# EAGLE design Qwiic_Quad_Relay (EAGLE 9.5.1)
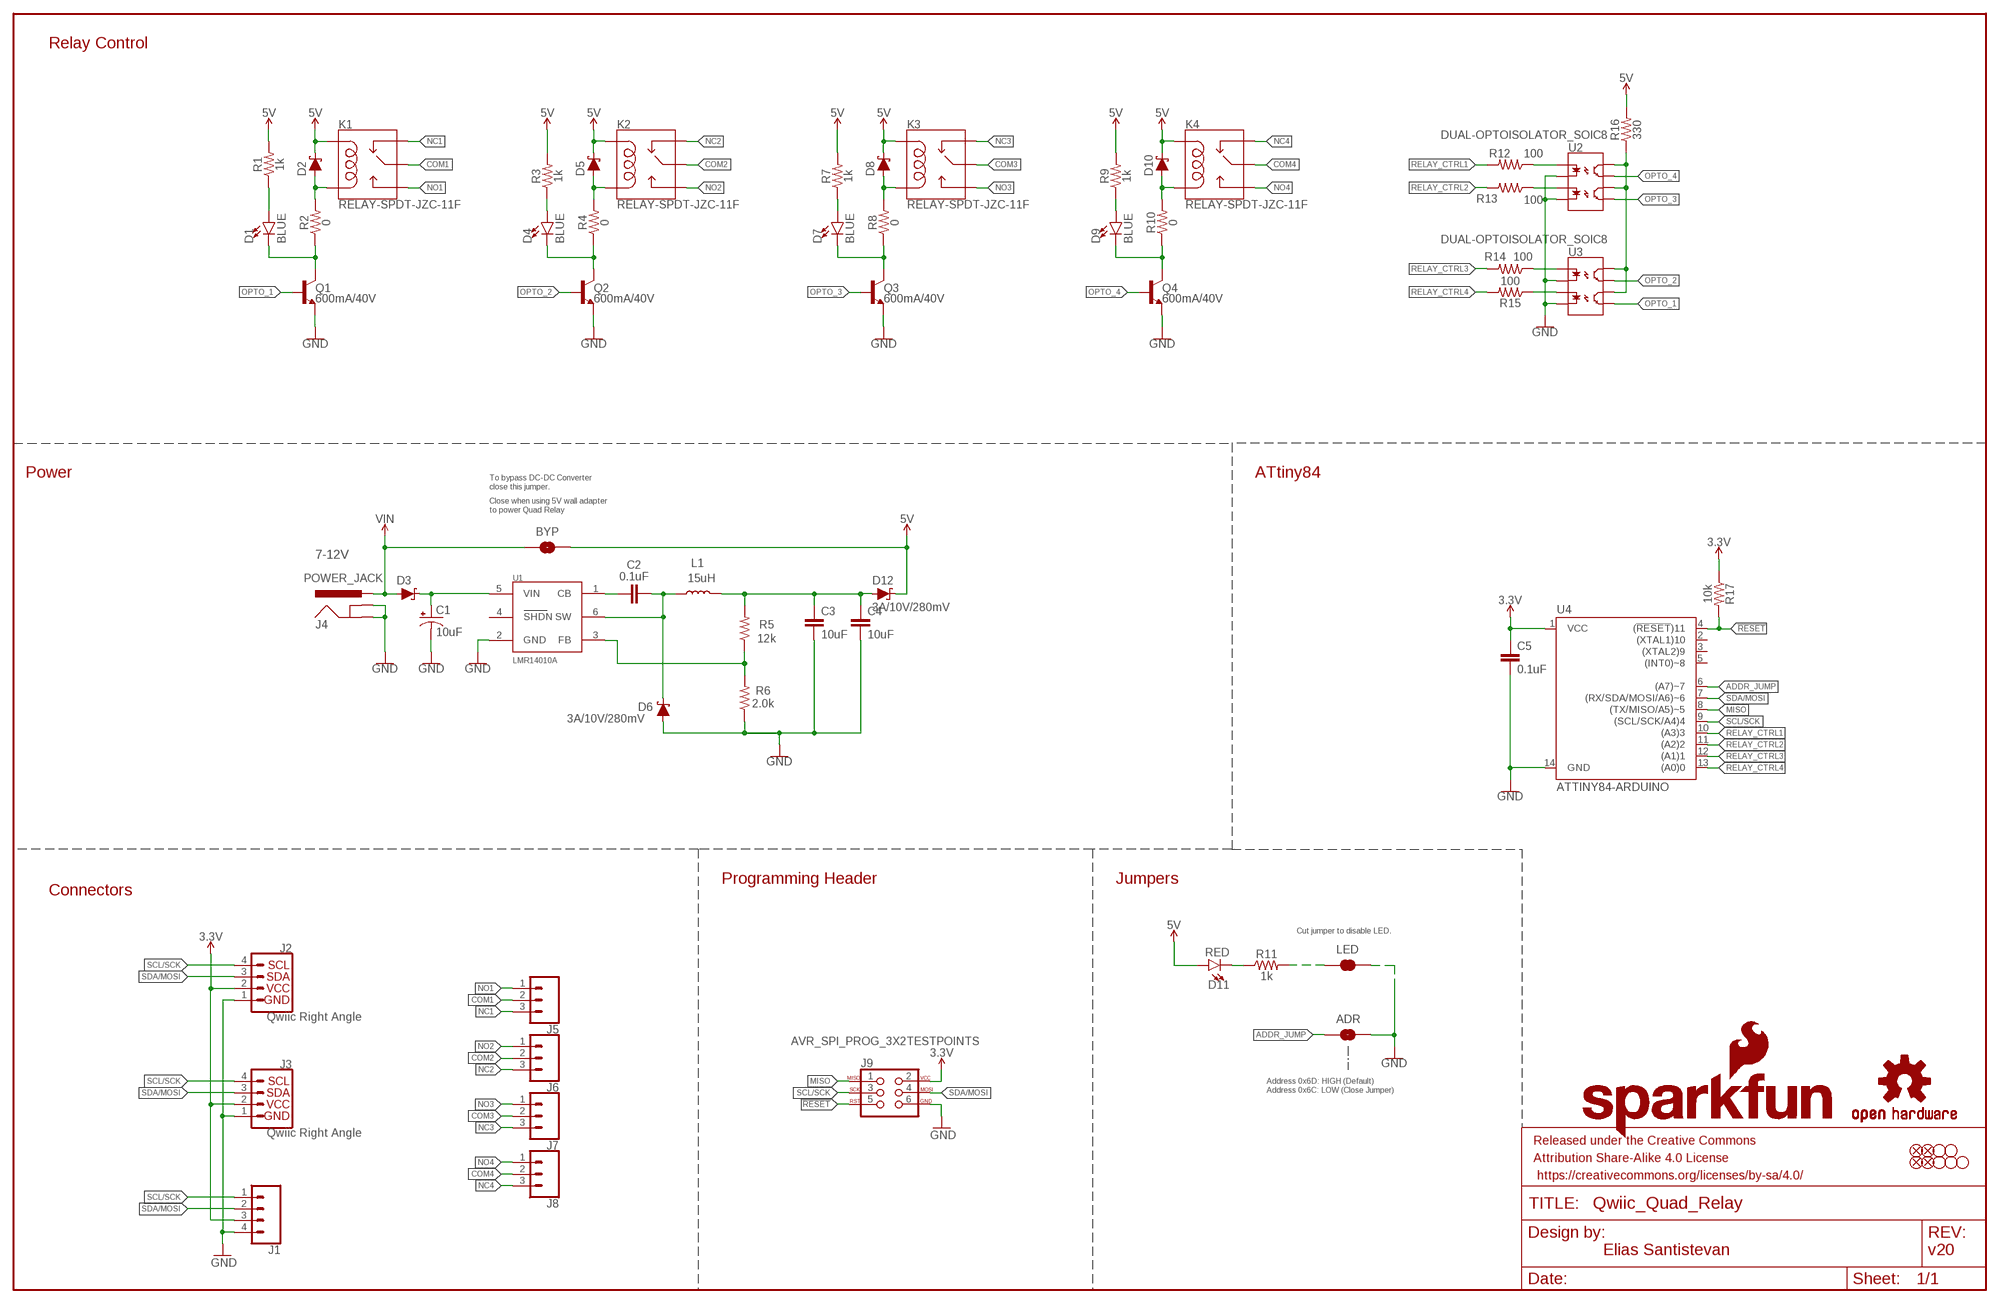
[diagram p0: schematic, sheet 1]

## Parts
ADR  JUMPER-SMT_2_NO_SILK  [SMT-JUMPER_2_NO_SILK]
BYP  JUMPER-SMT_2_NO_SILK  [SMT-JUMPER_2_NO_SILK]
C1  10uF  10UF-POLAR-EIA3528-20V-10%(TANT)  [EIA3528]
C2  0.1uF  0.1UF-0402-10V-10%-X7R  [0402]
C3  10uF  10UF-0603-6.3V-20%  [0603]
C4  10uF  10UF-0603-6.3V-20%  [0603]
C5  0.1uF  0.1UF-0603-25V-(+80/-20%)  [0603]
D1  BLUE  LED-BLUE0603  [LED-0603]
D2  1A/23V/620mV  DIODE-SCHOTTKY-BAT20J  [SOD-323]
D3  1A/40V/500mV  DIODE-SCHOTTKY-SS14  [SMA-DIODE]
D4  BLUE  LED-BLUE0603  [LED-0603]
D5  1A/23V/620mV  DIODE-SCHOTTKY-BAT20J  [SOD-323]
D6  3A/10V/280mV  DIODE-SCHOTTKY-BAT60A  [SOD-323]
D7  BLUE  LED-BLUE0603  [LED-0603]
D8  1A/23V/620mV  DIODE-SCHOTTKY-BAT20J  [SOD-323]
D9  BLUE  LED-BLUE0603  [LED-0603]
D10  1A/23V/620mV  DIODE-SCHOTTKY-BAT20J  [SOD-323]
D11  RED  LED-RED0603  [LED-0603]
D12  3A/10V/280mV  DIODE-SCHOTTKY-BAT60A  [SOD-323]
FD1  FIDUCIAL1X2  [FIDUCIAL-1X2]
FD2  FIDUCIAL1X2  [FIDUCIAL-1X2]
FD3  FIDUCIAL1X2  [FIDUCIAL-1X2]
FD4  FIDUCIAL1X2  [FIDUCIAL-1X2]
FRAME1  FRAME-LEDGER  [CREATIVE_COMMONS]
J1  CONN_041X04_NO_SILK_NO_POP  [1X04_NO_SILK]
J2  Qwiic Right Angle  I2C_STANDARDQWIIC  [JST04_1MM_RA]
J3  Qwiic Right Angle  I2C_STANDARDQWIIC  [JST04_1MM_RA]
J4  POWER_JACK  [POWER_JACK_PTH]
J5  CONN_03-SCREW-5MM  [SCREWTERMINAL-5MM-3]
J6  CONN_03-SCREW-5MM  [SCREWTERMINAL-5MM-3]
J7  CONN_03-SCREW-5MM  [SCREWTERMINAL-5MM-3]
J8  CONN_03-SCREW-5MM  [SCREWTERMINAL-5MM-3]
J9  AVR_SPI_PROG_3X2TESTPOINTS  [2X3_TEST_POINTS]
JP1  STAND-OFF  [STAND-OFF]
JP4  STAND-OFF  [STAND-OFF]
JP5  STAND-OFF  [STAND-OFF]
JP6  STAND-OFF  [STAND-OFF]
JP7  STAND-OFF  [STAND-OFF]
K1  RELAY-SPDT-JZC-11F  [RELAY-JZC]
K2  RELAY-SPDT-JZC-11F  [RELAY-JZC]
K3  RELAY-SPDT-JZC-11F  [RELAY-JZC]
K4  RELAY-SPDT-JZC-11F  [RELAY-JZC]
L1  15uH  INDUCTOR-LQH5B-15UH  [INDUCTOR_15UH]
LED  JUMPER-SMT_2_NC_TRACE_SILK  [SMT-JUMPER_2_NC_TRACE_SILK]
LOGO1  SFE_LOGO_NAME_FLAME.1_INCH  [SFE_LOGO_NAME_FLAME_.1]
LOGO2  OSHW-LOGOS  [OSHW-LOGO-S]
Q1  600mA/40V  TRANS_NPN-MMBT2222AL  [SOT23-3]
Q2  600mA/40V  TRANS_NPN-MMBT2222AL  [SOT23-3]
Q3  600mA/40V  TRANS_NPN-MMBT2222AL  [SOT23-3]
Q4  600mA/40V  TRANS_NPN-MMBT2222AL  [SOT23-3]
R1  1k  1KOHM-0603-1/10W-1%  [0603]
R2  0  0OHM-0603-1/10W  [0603]
R3  1k  1KOHM-0603-1/10W-1%  [0603]
R4  0  0OHM-0603-1/10W  [0603]
R5  12k  12KOHM-0603-1/10W-1%  [0603]
R6  2.0k  2.0KOHM-0603-1/10W-5%  [0603]
R7  1k  1KOHM-0603-1/10W-1%  [0603]
R8  0  0OHM-0603-1/10W  [0603]
R9  1k  1KOHM-0603-1/10W-1%  [0603]
R10  0  0OHM-0603-1/10W  [0603]
R11  1k  1KOHM-0603-1/10W-1%  [0603]
R12  100  100OHM-0603-1/10W-1%  [0603]
R13  100  100OHM-0603-1/10W-1%  [0603]
R14  100  100OHM-0603-1/10W-1%  [0603]
R15  100  100OHM-0603-1/10W-1%  [0603]
R16  330  330OHM-0603-1/10W-1%  [0603]
R17  10k  10KOHM-0603-1/10W-1%  [0603]
U1  LMR14010A  [SOT23-6]
U2  DUAL-OPTOISOLATOR_SOIC8  [SO08]
U3  DUAL-OPTOISOLATOR_SOIC8  [SO08]
U4  ATTINY84-ARDUINO  [SO14]

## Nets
3.3V: C5.1 J1.3 J2.2 J3.2 J9.2 R17.1 U4.1(VCC)
5V: BYP.2 D2.C D5.C D8.C D10.C D11.A D12.C K1.5(COIL1) K2.5(COIL1) K3.5(COIL1) K4.5(COIL1) R1.2 R3.2 R7.2 R9.2 R16.2
5V_OUT: C3.1 C4.1 D12.A L1.P2 R5.2
!RESET: J9.5 R17.2 U4.4((!RESET!)11)
ADDR_JUMP: ADR.1 U4.6((A7)~7)
CB: C2.1 U1.1(CB)
COM1: J5.2 K1.4(MAIN)
COM2: J6.2 K2.4(MAIN)
COM3: J7.2 K3.4(MAIN)
COM4: J8.2 K4.4(MAIN)
FB: R5.1 R6.2 U1.3(FB)
GND: ADR.2 C1.C(-) C3.2 C4.2 C5.2 D6.A J1.4 J2.1 J3.1 J4.GND J4.GNDBREAK J9.6 LED.1 Q1.2(E) Q2.2(E) Q3.2(E) Q4.2(E) R6.1 U1.2(GND) U2.2(C1) U2.4(C2) U3.2(C1) U3.4(C2) U4.14(GND)
MISO: J9.1 U4.8((TX/MISO/A5)~5)
N$1: D1.A R1.1
N$2: D1.C Q1.3(C) R2.1
N$3: R15.1 U3.3(A2)
N$4: D4.A R3.1
N$5: R14.1 U3.1(A1)
N$6: R16.1 U2.6(CL2) U2.8(CL1) U3.6(CL2) U3.8(CL1)
N$7: D7.A R7.1
N$8: D9.A R9.1
N$9: R12.1 U2.1(A1)
N$10: D2.A K1.1(COIL2) R2.2
N$11: R13.1 U2.3(A2)
N$12: D4.C Q2.3(C) R4.1
N$13: D11.C R11.1
N$14: LED.2 R11.2
N$15: D7.C Q3.3(C) R8.1
N$17: D9.C Q4.3(C) R10.1
N$18: D5.A K2.1(COIL2) R4.2
N$23: D8.A K3.1(COIL2) R8.2
N$24: D10.A K4.1(COIL2) R10.2
NC1: J5.3 K1.2(NC)
NC2: J6.3 K2.2(NC)
NC3: J7.3 K3.2(NC)
NC4: J8.3 K4.2(NC)
NO1: J5.1 K1.3(NO)
NO2: J6.1 K2.3(NO)
NO3: J7.1 K3.3(NO)
NO4: J8.1 K4.3(NO)
OPTO_1: Q1.1(B) U3.5(EM2)
OPTO_2: Q2.1(B) U3.7(EM1)
OPTO_3: Q3.1(B) U2.5(EM2)
OPTO_4: Q4.1(B) U2.7(EM1)
RELAY_CTRL1: R12.2 U4.10((A3)3)
RELAY_CTRL2: R13.2 U4.11((A2)2)
RELAY_CTRL3: R14.2 U4.12((A1)1)
RELAY_CTRL4: R15.2 U4.13((A0)0)
SCL/SCK: J1.1 J2.4 J3.4 J9.3 U4.9((SCL/SCK/A4)4)
SDA/MOSI: J1.2 J2.3 J3.3 J9.4 U4.7((RX/SDA/MOSI/A6)~6)
SW: C2.2 D6.C L1.P1 U1.6(SW)
VIN: BYP.1 D3.A J4.PWR
VIN_DC_DC: C1.A(+) D3.C U1.5(VIN)
Unconnected: U1.4(SHDN) U4.2((XTAL1)10) U4.3((XTAL2)9) U4.5((INT0)~8)

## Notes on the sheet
- Relay Control
- Power | ATtiny84
- To bypass DC-DC Converter
  close this jumper.
- Close when using 5V wall adapter
  to power Quad Relay
- 7-12V
- Programming Header | Jumpers
- Connectors
- Cut jumper to disable LED.
- Address 0x6D: HIGH (Default)
  Address 0x6C: LOW (Close Jumper)
- Elias Santistevan | v20

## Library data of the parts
ADR BYP = SparkFun-Jumpers:JUMPER-SMT_2_NO: Normally open jumper
C1 = SparkFun-Capacitors:10UF-POLAR: 10.0µF polarized capacitors; PROD_ID: CAP-08063
C2 = SparkFun-Capacitors:0.1UF: 0.1µF ceramic capacitors; PROD_ID: CAP-15083
C3 C4 = SparkFun-Capacitors:10UF: 10.0µF ceramic capacitors; PROD_ID: CAP-11015
C5 = SparkFun-Capacitors:0.1UF: 0.1µF ceramic capacitors; PROD_ID: CAP-00810
D1 D4 D7 D9 = SparkFun-LED:LED-BLUE: Blue SMD LED; PROD_ID: DIO-08575
D2 D5 D8 D10 = SparkFun-DiscreteSemi:DIODE-SCHOTTKY: Schottky diode; PROD_ID: DIO-11623
D3 = SparkFun-DiscreteSemi:DIODE-SCHOTTKY: Schottky diode; PROD_ID: DIO-08053
D6 D12 = SparkFun-DiscreteSemi:DIODE-SCHOTTKY: Schottky diode; PROD_ID: DIO-14072
D11 = SparkFun-LED:LED-RED: Red SMD LED; PROD_ID: DIO-00819
FD1-FD4 = SparkFun-Aesthetics:FIDUCIAL: Fiducial Alignment Points
FRAME1 = SparkFun-Aesthetics:FRAME-LEDGER: Schematic Frame - Ledger
J1 = SparkFun-Connectors:CONN_04: Multi connection point. Often used as Generic Header-pin footprint for 0.1 inch spaced/style header connections On any of the 0.1 inch spaced packages, you can populate with these: Break Away Headers - Straight (PRT-00116) Break Away Male Headers - Right Angle (PRT-00553) Female Headers (PRT-00115)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
J2 J3 = SparkFun-Connectors:I2C_STANDARD: SparkFun I2C Standard Pinout Header SparkFun has standardized on a pinout for all I2C based sensor breakouts. This pinout allows I2C boards to be plugged directly into the headers on Arduino Uno compatible boards, and to be daisy chained easily. Example SparkFun Products: SparkFun Atmospheric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; PROD_ID: CONN-13694
J4 = SparkFun-Connectors:POWER_JACK: Power Jack Connector This is the standard 5.5mm barrel jack for power. The PTH is the most common, proven, reliable, footprint. The Slot footprint only works if the mill layer is transmitted to the PCB fab house so be warned. Here are the connectors we sell at SparkFun: DC Barrel Power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; PROD_ID: CONN-08197
J5-J8 = SparkFun-Connectors:CONN_03: Multi connection point. Often used as Generic Header-pin footprint for 0.1 inch spaced/style header connections On any of the 0.1 inch spaced packages, you can populate with these: Break Away Headers - Straight (PRT-00116) Break Away Male Headers - Right Angle (PRT-00553) Female Headers (PRT-00115)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; PROD_ID: CONN-10134; SF_SKU: PRT-08433
J9 = SparkFun-Connectors:AVR_SPI_PROG_3X2: AVR ISP 6 Pin This is the reduced ISP connector for AVR programming. Common on Arduino. This footprint will take up less PCB space and can be used with a 10-pin to 6-pin adapter such as SKU: BOB-08508 **Special note about "TEST_POINT" package. The stop mask is on the top side, so if you want your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
JP1 JP4-JP7 = SparkFun-Hardware:STAND-OFF: Stand Off
K1-K4 = SparkFun-Electromechanical:RELAY-SPDT: SPDT Electromechanical Relay Single-pole, double-throw sealed relays. When current is applied to the coil, it throws a simple changeover switch, terminating the connection from the NC contact to ground and closing the NO contact. Use them to switch high voltage/high current devices. SparkFun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; PROD_ID: COMP-09533; SF_SKU: COM-00100
L1 = SparkFun-Coils:INDUCTOR: Inductors; PROD_ID: NDUC-15090
LED = SparkFun-Jumpers:JUMPER-SMT_2_NC_TRACE: Normally closed trace jumper
LOGO1 = SparkFun-Aesthetics:SFE_LOGO_NAME_FLAME: SparkFun Font Logo w/ Flame
LOGO2 = SparkFun-Aesthetics:OSHW-LOGO: Open-Source Hardware (OSHW) Logo
Q1-Q4 = SparkFun-DiscreteSemi:TRANS_NPN: NPN transistor Current controlled devices typically used to amplify current or used as a switch. BC547 - COM-08928 (TO-92 45V 100mA) (1.Collector 2.Base 3.Emitter) 2N3904 - COM-00521 (TO-92 40V 200mA) (1.Emitter 2.Base 3.Collector) P2N2222A - COM-12852 (TO-92 40V 600mA) (1.Collector 2.Base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; PROD_ID: TRANS-08049
R1 R3 R7 R9 R11 = SparkFun-Resistors:1KOHM: 1kΩ resistor; PROD_ID: RES-07856
R2 R4 R8 R10 = SparkFun-Resistors:0OHM: 0Ω resistor; PROD_ID: RES-08609
R5 = SparkFun-Resistors:12KOHM: 12kΩ resistor; PROD_ID: RES-10327
R6 = SparkFun-Resistors:2.0KOHM: 2kΩ resistor; PROD_ID: RES-08296
R12-R15 = SparkFun-Resistors:100OHM: 100Ω resistor; PROD_ID: RES-07863
R16 = SparkFun-Resistors:330OHM: 330Ω resistor; PROD_ID: RES-00818
R17 = SparkFun-Resistors:10KOHM: 10kΩ resistor; PROD_ID: RES-00824
U1 = SparkFun-IC-Power:LMR14010A: LMR14010A Buck Regulator 1A Output The LMR14010A is a PWM DC-to-DC buck (stepdown) regulator. With a wide input range from 4 V to 40 V, it is suitable for a wide range of applications from industrial to automotive. An ultra-low 1-µA shutdown current prolongs battery life. Operating frequency is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; PROD_ID: IC-15089
U2 U3 = SparkFun-DiscreteSemi:DUAL-OPTOISOLATOR: Optocoupler, Phototransistor Output, Dual Channel Optically coupled pairs with a gallium arsenide infrared LED and a silicon NPN phototransistor. Signal information, including a DC level, can be transmitted by the device while maintaining a high degree of electrical isolation between input and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; PROD_ID: IC-09076
U4 = SparkFun-IC-Microcontroller:ATTINY84-ARDUINO; PROD_ID: IC-14155

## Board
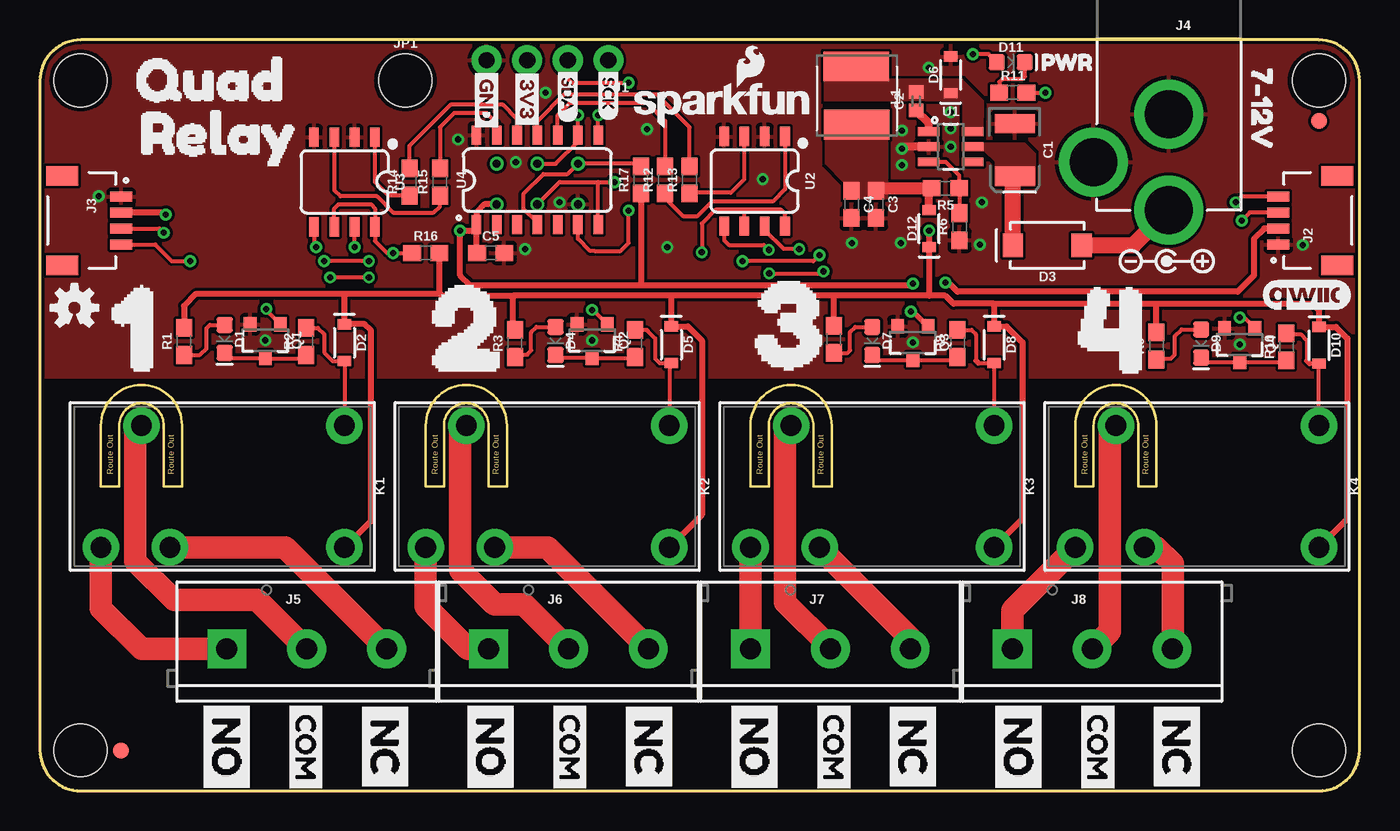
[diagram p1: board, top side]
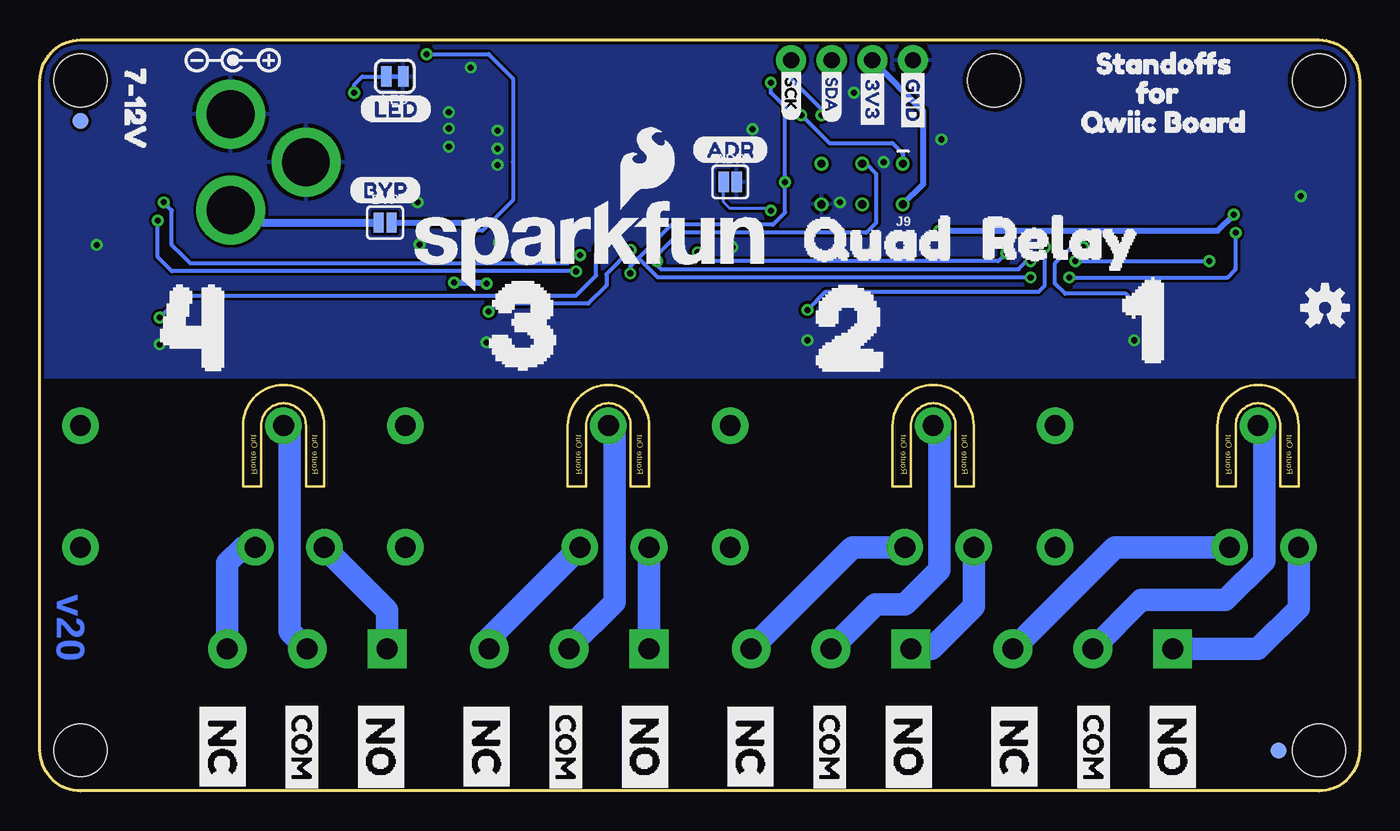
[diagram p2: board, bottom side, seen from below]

Size 82.55 x 46.99 mm. Coordinates in mm from the lower left corner, seen from the top.
Outline: 80.01,46.99 2.54,46.99 arc90 0,44.45 0,2.54 arc90 2.54,0 80.01,0 arc90 82.55,2.54 82.55,44.45 arc90 80.01,46.99
Outline: 28.07,19.05 28.07,22.86 arc90 26.67,24.26 arc90 25.27,22.86 25.27,19.05 24.13,19.05 24.13,22.86 arc-90 26.67,25.4 arc-90 29.21,22.86 29.21,19.05 28.07,19.05
Outline: 7.75,19.05 7.75,22.86 arc90 6.35,24.26 arc90 4.95,22.86 4.95,19.05 3.81,19.05 3.81,22.86 arc-90 6.35,25.4 arc-90 8.89,22.86 8.89,19.05 7.75,19.05
Outline: 48.39,19.05 48.39,22.86 arc90 46.99,24.26 arc90 45.59,22.86 45.59,19.05 44.45,19.05 44.45,22.86 arc-90 46.99,25.4 arc-90 49.53,22.86 49.53,19.05 48.39,19.05
Outline: 68.71,19.05 68.71,22.86 arc90 67.31,24.26 arc90 65.91,22.86 65.91,19.05 64.77,19.05 64.77,22.86 arc-90 67.31,25.4 arc-90 69.85,22.86 69.85,19.05 68.71,19.05
Copper layers (1*16): Top 0.035mm / dielectric 1.5mm / Bottom 0.035mm
Design rules "SparkFun-2-layer-TIGHT": minimum track width 7mil, minimum drill 15mil, track to track 7mil, track to pad 7mil, pad to pad 7mil, via to via 7mil, smd to smd 7mil, copper to edge 7mil, drill to drill 7mil, minimum pad ring 7mil, minimum via ring 7mil, stop-mask expansion 4mil, vias tented up to drill 25mil, thermal gap 10mil

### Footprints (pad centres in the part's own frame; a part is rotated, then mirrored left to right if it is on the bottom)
SMT-JUMPER_2_NO_SILK = smd 0.635 x 1.27: 1 -0.406,0; 2 0.406,0
EIA3528 = smd 1.2 x 2.5: A 1.65,0; C -1.65,0
0402 = smd 0.85 x 0.9: 1 -0.58,0; 2 0.58,0
0603 = smd 1.1 x 1: 1 -0.85,0; 2 0.85,0
LED-0603 = smd 1 x 1: A -0.877,0; C 0.877,0
SOD-323 = smd 0.63 x 0.83: A 1.15,0; C -1.15,0
SMA-DIODE = smd 1.27 x 1.47: A -2.15,0; C 2.15,0
FIDUCIAL-1X2 = smd 1 x 1: 1 0,0
1X04_NO_SILK = drill 1.016 pad 1.88: 1 0,0; 2 2.54,0; 3 5.08,0; 4 7.62,0
JST04_1MM_RA = smd 0.6 x 1.35: 1 -1.5,0; 2 -0.5,0; 3 0.5,0; 4 1.5,0 | smd 1.2 x 2: NC1 2.8,-3.675; NC2 -2.8,-3.675
POWER_JACK_PTH = drill 2.997 pad 4.318: GND 0,7.7; GNDBREAK 4.7,10.7; PWR 0,13.7
SCREWTERMINAL-5MM-3 = drill 1.3 pad 2.413 square: 1 0,0 | drill 1.3 pad 2.413: 2 5,0; 3 10,0
2X3_TEST_POINTS = drill 0.508: 1 -2.54,-1.27; 2 -2.54,1.27; 3 0,-1.27; 4 0,1.27; 5 2.54,-1.27; 6 2.54,1.27
STAND-OFF = hole 3.302: 0,0
RELAY-JZC = drill 1.3 pad 2.286: 1 3.81,-8.89; 2 -3.81,2.032; 3 -3.81,6.35; 4 3.81,3.81; 5 -3.81,-8.89
INDUCTOR_15UH = smd 1.85 x 4.1: P1 -1.905,0; P2 1.745,0.05
SMT-JUMPER_2_NC_TRACE_SILK = smd 0.66 x 1.27: 1 -0.521,0; 2 0.521,0
SOT23-3 = smd 0.8 x 0.9: 1 -0.95,-1; 2 0.95,-1; 3 0,1.1
SOT23-6 = smd 0.55 x 1.35: 1 -0.95,-1.375; 2 0,-1.375; 3 0.95,-1.375; 4 0.95,1.375; 5 0,1.375; 6 -0.95,1.375
SO08 = smd 0.6 x 1.2: 1 -1.905,-2.8; 2 -0.635,-2.8; 3 0.635,-2.8; 4 1.905,-2.8; 5 1.905,2.8; 6 0.635,2.8; 7 -0.635,2.8; 8 -1.905,2.8
SO14 = smd 0.6 x 1.2: 1 -3.81,-2.8; 2 -2.54,-2.8; 3 -1.27,-2.8; 4 0,-2.8; 5 1.27,-2.8; 6 2.54,-2.8; 7 3.81,-2.8; 8 3.81,2.8; 9 2.54,2.8; 10 1.27,2.8; 11 0,2.8; 12 -1.27,2.8; 13 -2.54,2.8; 14 -3.81,2.8

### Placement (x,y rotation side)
ADR  39.37,38.1 0 bottom
BYP  60.96,35.56 0 bottom
C1  60.99,40.11 270 top
C2  54.81,43.15 90 top
C3  52.3,36.7 270 top
C4  50.77,36.7 270 top
C5  28.19,33.66 0 top
D1  11.56,28.28 270 top
D2  19.05,28.05 270 top
D3  63.02,34.14 180 top
D4  32.26,28.16 270 top
D5  39.5,27.92 270 top
D6  56.97,44.81 90 top
D7  52.07,28.16 270 top
D8  59.69,27.92 270 top
D9  72.64,28 270 top
D10  80.01,27.89 270 top
D11  60.73,45.59 0 top
D12  55.63,35.18 90 top
FD1  80.01,41.91 0 bottom
FD2  5.08,2.54 0 top
FD3  5.08,2.54 0 bottom
FD4  80.01,41.91 0 top
FRAME1  not placed on the board
J1  35.56,45.72 180 top
J2  77.47,35.69 90 top
J3  5.08,35.69 270 top
J4  70.61,50.04 180 top
J5  11.68,8.89 0 top
J6  28.07,8.89 0 top
J7  44.45,8.89 0 top
J8  60.83,8.89 0 top
J9  31.11,37.97 180 bottom
JP1  22.86,44.45 0 top
JP4  2.54,44.45 0 top
JP5  80.01,44.45 0 top
JP6  2.54,2.54 0 top
JP7  80.01,2.54 0 top
K1  10.16,19.05 90 top
K2  30.48,19.05 90 top
K3  50.8,19.05 90 top
K4  71.12,19.05 90 top
L1  51.05,43.43 270 top
LED  60.35,44.7 180 bottom
LOGO1  42.72,42.93 0 top
LOGO2  2.16,30.23 0 top
Q1  14.1,28.19 180 top
Q2  34.54,28.19 180 top
Q3  54.61,28.07 180 top
Q4  75.06,27.94 180 top
R1  9.02,28.13 90 top
R2  16.64,28.13 90 top
R3  29.72,28 90 top
R4  37.21,28 90 top
R5  56.64,37.72 180 top
R6  57.53,35.31 90 top
R7  49.66,28.25 90 top
R8  57.4,28 90 top
R9  69.85,27.84 90 top
R10  77.98,27.78 90 top
R11  60.86,43.69 0 top
R12  39.12,38.23 90 top
R13  40.64,38.23 90 top
R14  23.11,38.1 90 top
R15  25.02,38.1 90 top
R16  24.13,33.66 0 top
R17  37.59,38.23 90 top
U1  56.97,40.31 270 top
U2  44.7,38.15 180 top
U3  19.05,38.1 180 top
U4  31.11,38.23 0 top
U$1  [7#12V0]  76.45,46.35 270 top
U$2  [20]  19.94,28.96 0 top
U$3  [10]  -0.13,28.96 0 top
U$4  [30]  40.13,29.21 0 top
U$5  [40]  60.33,28.83 0 top
U$6  [QUAD0]  3.66,44.5 0 top
U$7  [RELAY0]  4.04,41.15 0 top
U$8  [SCK-[)-03]  35.56,45.34 270 top
U$9  [GND-03]  27.94,45.34 270 top
U$10  [3V3-03]  30.48,45.34 270 top
U$11  [SDA0]  33.02,45.34 270 top
U$12  [3V3-03]  30.48,45.34 270 bottom
U$13  [OSHW-LOGO-S]  2.16,30.23 0 bottom
U$14  [BYP]  63.25,37.59 0 bottom
U$15  [NO0]  11.68,6.22 270 top
U$16  [COM0]  16.64,5.97 270 top
U$17  [NC0]  21.59,6.1 270 top
U$18  [NO0]  28.19,6.22 270 top
U$19  [COM0]  33.15,5.97 270 top
U$20  [NC0]  38.1,6.1 270 top
U$21  [NO0]  44.7,6.22 270 top
U$22  [COM0]  49.66,5.97 270 top
U$23  [NC0]  54.61,6.1 270 top
U$24  [NO0]  61.21,6.22 270 top
U$25  [COM0]  66.17,5.97 270 top
U$26  [NC0]  71.12,6.1 270 top
U$27  [NO0]  44.7,6.22 270 bottom
U$28  [COM0]  66.17,5.97 270 bottom
U$29  [NC0]  71.12,6.1 270 bottom
U$30  [NO0]  61.21,6.22 270 bottom
U$31  [COM0]  49.66,5.97 270 bottom
U$32  [NC0]  54.61,6.1 270 bottom
U$33  [NO0]  28.19,6.22 270 bottom
U$34  [COM0]  33.15,5.97 270 bottom
U$35  [NC0]  38.1,6.1 270 bottom
U$36  [NO0]  11.68,6.22 270 bottom
U$37  [COM0]  16.64,5.97 270 bottom
U$38  [NC0]  21.59,6.1 270 bottom
U$39  [10]  19.43,29.46 0 bottom
U$40  [20]  38.61,28.96 0 bottom
U$41  [30]  59.05,29.21 0 bottom
U$42  [40]  79.63,28.99 0 bottom
U$43  [QUAD0]  37.13,34.54 0 bottom
U$44  [RELAY0]  25.86,34.59 0 bottom
U$45  [GND-03]  27.94,45.34 270 bottom
U$46  [PWR_TO]  61.72,45.59 0 top
U$47  [SDA0]  33.02,45.34 270 bottom
U$48  [SCK-[)-03]  35.56,45.34 270 bottom
U$49  [7#12V0]  76.58,46.35 270 bottom
U$50  [STANDOFFS0]  17.63,45.52 0 bottom
U$51  [POLARITY_MARKING_CENTER_POSITIVE#JPG]  70.48,33.15 0 top
U$52  [FOR1]  15.14,43.69 0 bottom
U$53  [LED]  62.59,42.67 0 bottom
U$54  [POLARITY_MARKING_CENTER_POSITIVE#JPG]  70.48,45.72 0 bottom
U$55  [QWIIC_5.5MM]  79.25,31.04 0 top
U$56  [ADR-()-04]  41.78,40.13 0 bottom
U$57  [SFE_LOGO_NAME_FLAME_.2]  48.11,34.14 0 bottom
U$58  [QWIIC_BOARD2]  18.54,41.86 0 bottom

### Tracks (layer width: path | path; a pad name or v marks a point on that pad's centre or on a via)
3.3V  (via drill 0.38)
  Top 0.381: J2.2 76.59,35.19 75.95,34.54 75.95,32.26 74.93,31.24 57.4,31.24 56.84,31.8 v56.64,31.8 | v54.61,31.75 54.48,31.62 37.59,31.62 | R17.1 37.59,31.62 | 37.59,31.62 26.92,31.62 26.29,32.26 v26.29,35.05 27.3,35.05 | J9.2 27.81,36.7 27.3,36.2 U4.1 27.3,35.05 | C5.1 27.3,33.69 27.3,35.05 | v7.87,36.07 7.75,36.19 J3.2
  Bottom 0.381: v7.87,36.07 8.89,35.05 v26.29,35.05 | J9.2 28.55,36.7 27.3,37.95 27.3,42.55 J1.3 | v56.64,31.8 54.66,31.8 v54.61,31.75
5V  (via drill 0.38)
  Top 0.254: v58.37,46.1 59.35,46.1 D11.A
  Top 0.381: 49.66,30.99 39.5,30.99 | 39.5,30.99 29.59,30.99 | 59.69,30.48 57.15,30.48 56.64,30.99 55.63,30.99 | 19.05,31.11 9.78,31.11 9.02,30.35 R1.2 | 19.05,31.11 25.02,31.11 | 29.59,30.99 25.15,30.99 25.02,31.11 | D2.C | D2.C 19.05,31.11 | K1.5 20.7,16.89 20.7,28.83 20.32,29.21 D2.C | 59.69,30.48 D8.C 60.46,29.07 61.47,28.07 61.47,17.02 K3.5 | 39.5,30.99 D5.C 40.52,29.07 41.4,28.19 41.4,17.27 K2.5 | R7.2 49.66,30.99 | 59.69,30.48 69.85,30.48 | 69.85,30.48 79.63,30.48 80.01,30.1 D10.C 81.07,29.04 81.79,28.32 81.79,17.02 K4.5 | R9.2 69.85,30.48 | R16.2 24.98,31.15 25.02,31.11 | R3.2 29.59,28.98 29.59,30.99 | 55.63,30.99 49.66,30.99 | 55.63,30.99 D12.C v55.63,35.05
  Bottom 0.254: v58.37,46.1 54.48,46.1 52.96,44.58 52.96,39.37 52.96,36.96 54.86,35.05 v55.63,35.05
  Bottom 0.381: BYP.2 56.13,35.56 v55.63,35.05
5V_OUT
  Top 0.508: D12.A 55.63,37.55 R5.2
  Top 0.762: R5.2 55.75,37.68 52.43,37.68 C3.1
  pour Top (isolate 0.305, no thermals): 49.12,42.55 49.12,39.27 50.29,38.1 50.29,37.08 53.01,37.08 53.01,42.55
!RESET
  Top 0.254: R17.2 37.43,39.24 J9.5 33.02,38.61 31.5,38.61 30.23,37.34 30.23,36.44 31.11,35.55 U4.4
ADDR_JUMP  (via drill 0.38)
  Top 0.254: U4.6 33.66,34.54 34.42,33.78 34.69,33.78 36.32,33.78 36.83,34.29 v36.83,36.32
  Bottom 0.203: v36.83,36.32 36.96,36.45 39.37,36.45 39.78,36.85 ADR.1
CB
  Top 0.508: U1.1 55.6,41.79 C2.1
COM1
  Top 1.397: J5.2 16.64,8.89 13.59,11.94 8.89,11.94 8.38,11.94 5.97,14.35 5.97,22.48 K1.4
  Bottom 1.397: J5.2 13.64,11.94 8.38,11.94 5.97,14.35 5.97,22.48 K1.4
COM2
  Top 1.397: J6.2 30.27,11.68 28.45,11.68 26.29,13.84 26.29,22.48 K2.4
  Bottom 1.397: J6.2 30.27,11.68 28.45,11.68 26.29,13.84 26.29,22.48 K2.4 | J6.2
COM3
  Top 1.397: J7.2 49.45,8.97 46.61,11.81 46.61,22.48 K3.4
  Bottom 1.397: J7.2 49.45,8.97 46.61,11.81 46.61,22.48 K3.4
COM4
  Top 1.397: K4.4 66.93,22.48 66.93,9.99 J8.2
  Bottom 1.397: K4.4 66.93,22.48 66.93,9.99 J8.2
FB
  Top 0.254: U1.3 56.65,39.36 57.49,38.52 R5.1 57.53,37.68 R6.2
GND  (via drill 0.38)
  Top 0.508: U1.2 54.05,40.31 v53.92,40.18
  other vias: 30.35,33.91 39.24,34.04 37.97,41.4 50.8,34.29 45.21,38.28 31.62,43.69 29.77,39.34 26.16,40.77 32.51,36.83 34.54,28.19 14.1,28.19 54.61,28.07 75.06,27.94 53.92,39.17 58.8,34.19 55.6,45.26 78.99,34.16 3.68,37.21 53.85,34.29 58.93,36.83 56.97,40.31 56.97,41.45 56.97,42.47 53.92,41.33
  pour Bottom (rank 2): 0,25.91 82.55,25.91 82.55,46.99 0,46.99
  pour Top (rank 2): 0,25.91 0,46.99 82.55,46.99 82.55,25.91
MISO  (via drill 0.38)
  Top 0.254: U4.8 v34.92,42.29
  Bottom 0.254: v34.92,42.29 33.17,40.54 29.23,40.54 28.57,39.88 J9.1
N$1
  Top 0.254: R1.1 10.01,27.28 10.41,27.69 10.41,28.96 10.62,29.16 D1.A
N$2
  Top 0.254: R2.1 16.41,27.05 14.14,27.05 Q1.3 11.87,27.09 D1.C
N$3
  Top 0.254: U3.3 18.41,37.59 18.8,37.21 21.08,37.21 22.1,36.2 24.64,36.2 25.02,36.58 R15.1
N$4
  Top 0.254: R3.1 29.87,27.3 30.48,27.3 30.73,27.56 30.73,28.7 31.07,29.03 D4.A
N$5
  Top 0.254: R14.1 21.8,37.25 20.95,38.1 U3.1
N$6  (via drill 0.38)
  Top 0.254: U3.6 18.41,36.45 18.67,36.7 20.7,36.7 20.95,36.45 U3.8 20.95,34.42 21.72,33.66 v22.1,33.66 R16.1 | 44.07,36.37 46.35,36.37 46.61,36.12 U2.8 | U2.6 44.07,36.37 | 44.07,36.37 42.27,36.37 41.4,35.51 v41.4,33.71
  Bottom 0.254: v41.4,33.71 40.84,33.15 22.61,33.15 v22.1,33.66
N$7
  Top 0.254: D7.A 51,29.03 50.67,28.7 50.67,27.56 50.52,27.4 R7.1
N$8
  Top 0.254: 69.91,27.05 70.74,27.05 70.99,27.3 70.99,28.45 71.42,28.88 D9.A
  Top 0.305: R9.1 69.91,27.05
N$9
  Top 0.254: U2.1 46.61,37.64 45.85,36.88 42.04,36.88 41.1,35.94 40.26,35.94 39.12,37.08 R12.1
N$10
  Top 0.254: R2.2 17.38,28.98 17.78,28.57 | 17.78,28.57 | 17.78,28.57 17.78,27.43 18.31,26.9 D2.A K1.1
N$11
  Top 0.254: U2.3 44.07,38.28 43.22,37.43 40.69,37.43 R13.1
N$12
  Top 0.254: D4.C 32.44,27.09 Q2.3 37.16,27.09 R4.1
N$13
  Top 0.254: D11.C 61.62,44.7 61.49,44.58 60.22,44.58 60.01,44.36 R11.1
N$14  (via drill 0.38)
  Top 0.254: R11.2 v62.89,43.69
  Bottom 0.254: v62.89,43.69 62.89,44.2 62.38,44.7 LED.2
N$15
  Top 0.254: 52.38,26.97 Q3.3 57.22,26.97
  Top 0.305: D7.C 52.38,26.97 | 57.22,26.97 R8.1
N$17
  Top 0.254: 72.92,26.84 Q4.3 77.88,26.84
  Top 0.305: D9.C 72.92,26.84 | 77.88,26.84 R10.1
N$18
  Top 0.254: K2.1 39.37,26.64 D5.A 38.76,26.77 38.48,27.05 38.48,28.32 38.01,28.79 37.95,28.85 R4.2
N$23
  Top 0.254: R8.2 58.27,28.85 58.55,28.57 58.55,26.92 | 58.7,26.77 D8.A K3.1
  Top 0.305: 58.55,26.92 58.7,26.77
N$24
  Top 0.254: 78.04,28.57 78.87,28.57 79.25,28.19 79.25,26.92 | 79.43,26.74 D10.A K4.1
  Top 0.305: R10.2 78.04,28.57 | 79.25,26.92 79.43,26.74
NC1
  Top 1.397: K1.2 15.33,15.24 J5.3
  Bottom 1.397: K1.2 15.32,15.24 21.67,8.89 J5.3
NC2
  Top 1.397: K2.2 31.75,15.24 38.07,8.92 J6.3
  Bottom 1.397: K2.2 31.72,15.24 J6.3
NC3
  Top 1.397: J7.3 54.45,9.56 K3.2
  Bottom 1.397: 54.48,8.89 54.48,9.53 K3.2
NC4
  Top 1.397: J8.3 70.87,8.92 70.87,14.22 69.85,15.24 K4.2
  Bottom 1.397: J8.3 70.83,13.97 70.83,14.26 69.85,15.24 K4.2
NO1
  Top 1.397: K1.3 3.81,11.43 6.35,8.89 J5.1
  Bottom 1.397: J5.1 6.35,8.89 3.81,11.43 K1.3
NO2
  Top 1.397: J6.1 26.8,8.89 24.13,11.56 K2.3
  Bottom 1.397: J6.1 26.8,8.89 24.13,11.56 K2.3
NO3
  Top 1.397: J7.1 K3.3
  Bottom 1.397: J7.1 K3.3
NO4
  Top 1.397: J8.1 60.83,11.3 K4.3
  Bottom 1.397: J8.1 60.83,11.3 K4.3
OPTO_1  (via drill 0.38)
  Top 0.254: U3.5 17.14,34.16 v17.27,34.04 | Q1.1 14.16,30.08 v14.16,30.16
  Bottom 0.254: v17.27,34.04 18.03,34.04 19.05,33.02 19.05,31.75 18.41,31.11 14.61,31.11 14.16,30.67 v14.16,30.16
OPTO_2  (via drill 0.38)
  Top 0.254: v19.68,34.04 U3.7 | v34.54,30.1 34.59,30.1 Q2.1
  Bottom 0.254: v19.68,34.04 19.68,31.62 20.07,31.24 33.4,31.24 v34.54,30.1
OPTO_3  (via drill 0.38)
  Top 0.254: U2.5 42.8,34.47 43.1,34.16 45.29,34.16 v45.59,33.86
  Top 0.305: Q3.1 55.54,29.07 54.61,30 v54.48,30
  Bottom 0.254: v45.59,33.86 47.12,32.33 47.12,31.62 48.26,30.48 54,30.48 v54.48,30
OPTO_4  (via drill 0.38)
  Top 0.254: v47.5,33.91 46.53,33.91 45.34,35.1 U2.7 | v75.05,29.62 75.33,29.62 Q4.1
  Bottom 0.254: v47.5,33.91 47.75,33.66 47.75,32.26 49.02,30.99 73.68,30.99 v75.05,29.62
RELAY_CTRL1
  Top 0.254: R12.2 39.12,41.91 37.97,43.05 33.15,43.05 32.38,42.29 U4.10
RELAY_CTRL2
  Top 0.254: U4.11 | U4.11 31.11,41.91 32.77,43.56 36.07,43.56 | 36.07,43.56 38.61,43.56 40.64,41.53 R13.2 | 36.07,43.56
RELAY_CTRL3
  Top 0.254: R14.2 23.11,40.36 25.68,42.93 28.96,42.93 29.84,42.04 U4.12
RELAY_CTRL4
  Top 0.254: R15.2 25.02,41.53 25.91,42.42 27.94,42.42 28.57,41.78 U4.13
SCL/SCK  (via drill 0.38)
  Top 0.254: J2.4 75.16,37.19 v74.8,36.83 | v43.94,33.15 48.39,33.15 v48.77,33.53 | v20.57,33.15 v17.78,33.15 | J3.4 7.21,34.19 8.26,33.15 v9.4,33.15 | v33.66,42.29 U4.9 33.66,40.64 32.26,39.24 J9.3
  Bottom 0.254: v17.78,33.15 v9.4,33.15 | J1.1 35.56,44.58 33.66,42.67 v33.66,42.29 | J9.3 30.86,39.24 30.23,38.61 30.23,35.56 30.86,34.92 42.55,34.92 43.94,33.53 v43.94,33.15 43.94,32.89 43.69,32.64 21.34,32.64 20.83,33.15 v20.57,33.15 | v74.8,36.83 74.3,36.32 74.3,34.16 73.66,33.53 73.15,33.02 49.53,33.02 49.02,33.53 v48.77,33.53 | v20.57,33.15
SDA/MOSI  (via drill 0.38)
  Top 0.254: v20.57,32.13 v18.16,32.13 | J1.2 33.02,44.58 33.27,44.32 v36.83,44.32 | J9.4 32.51,38.1 34.92,38.1 | 34.92,38.1 v35.94,38.1 | J3.3 7.49,35.19 v7.75,34.92 | v75.18,35.69 75.68,36.19 J2.3 | v49.02,32.51 48.9,32.38 v45.62,32.38 | U4.7 34.92,38.1
  Bottom 0.254: v18.16,32.13 8.26,32.13 7.75,32.64 v7.75,34.92 | v35.94,38.1 35.94,36.2 36.7,35.43 43.03,35.43 45.11,33.35 | v35.94,38.1 | v35.94,38.1 35.94,42.8 36.83,43.69 v36.83,44.32 | v75.18,35.69 75.18,33.4 74.3,32.51 v49.02,32.51 | v20.57,32.13 43.89,32.13 45.11,33.35 | v45.62,32.38 45.62,32.84 45.11,33.35
SW
  pour Top (no thermals): 57.73,41.07 58.98,41.07 59.02,43.17 57.68,44.51 52.93,44.51 52.93,46.18 49.07,46.18 49.07,43.21 57.73,43.21
VIN
  Top 1.016: D3.A 68.41,34.14 J4.PWR
  Bottom 0.508: BYP.1 69.83,35.56 J4.PWR
VIN_DC_DC
  Top 1.016: D3.C 60.87,38.34 C1.A
  pour Top (no thermals): 62.23,39.88 62.23,37.9 59.79,37.9 59.79,39.37 59.13,40.04 57.73,40.06 57.73,40.54 61.57,40.54

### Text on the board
Bottom: v20
Dimension: Route Out | Route Out | Route Out | Route Out | Route Out | Route Out | Route Out | Route Out
tDocu: Elias Santistevan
